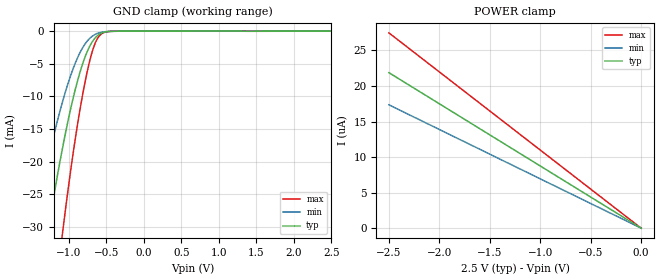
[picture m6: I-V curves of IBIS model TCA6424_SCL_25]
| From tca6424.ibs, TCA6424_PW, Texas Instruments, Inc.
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[Model]   TCA6424_SCL_25
Model_type  Input
Vinl=0.69
Vinh=1.89
| variable   typ   min   max
C_comp   2.19pF   1.68pF   2.42pF
[Temperature Range]   40   100   -40
| Ambient temperature   25   85   -40
[Voltage range]   2.5   2.3   2.7
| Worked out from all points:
|   GND clamp passes 1 mA (typ) near -0.65 V on its own axis
[GND Clamp]
| TCA6424_SCL_25
|   Voltage   I(typ)   I(min)   I(max)
-2.5V     -143.4mA   -105mA     -204.1mA
-1.49V    -47.01mA   -31.58mA   -73.96mA
-1.46V    -44.57mA   -29.8mA    -70.48mA
-1.27V    -30.12mA   -19.36mA   -49.42mA
-1.085V   -17.96mA   -10.85mA   -30.98mA
-955mV    -10.86mA   -6.127mA   -19.7mA
-840mV    -5.87mA    -3.043mA   -11.28mA
-730mV    -2.509mA   -1.205mA   -4.961mA
-650mV    -1.053mA   -502.7uA   -1.883mA
-560mV    -279.8uA   -153.1uA   -377.5uA
-440mV    -30.06uA   -22.66uA   -28.84uA
2.5V      205.9pA    1.388uA    -2.198uA
[POWER Clamp]
| TCA6424_SCL_25
|   Voltage   I(typ)   I(min)   I(max)
-2.5V     21.87uA    17.35uA    27.47uA
-1.535V   13.43uA    10.65uA    16.87uA
-1.145V   10.02uA    7.946uA    12.58uA
-31.15fV  205.9pA    679.2pA    48.94pA
